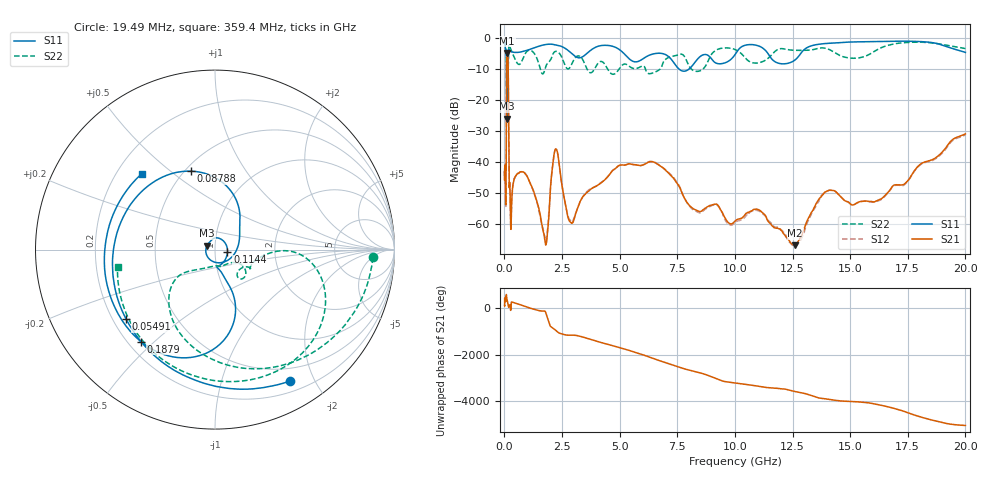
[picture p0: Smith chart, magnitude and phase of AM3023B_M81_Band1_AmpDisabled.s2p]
!Agilent Technologies,E8364B,MY43040894,A.07.50.67
!Agilent E8364B: A.07.50.67
!Date: Tuesday, October 27, 2020 10:39:40
!Correction: S11(Full 2 Port(1,2))
!S21(Full 2 Port(1,2))
!S12(Full 2 Port(1,2))
!S22(Full 2 Port(1,2))
!S2P File: Measurements: S11, S21, S12, S22:Log Frequency Sweep
# Hz S  dB  R 50
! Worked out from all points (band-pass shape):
!   3201 points, 10 MHz to 20 GHz, reference 50 ohm
!   highest |S21| = -4.93 dB at 122.5 MHz (marker M1); lowest = -66.9 dB at 12.62 GHz (marker M2)
!   |S21| within 3 dB of the highest: 96.52 MHz to 162.3 MHz (65.75 MHz wide, 50.8 % of centre)
!   lowest |S11| = -26.1 dB at 102.6 MHz (marker M3), VSWR 1.10, Z = 45.7 + j1.99 ohm
!   |S11| at or under -10 dB: 91.5 MHz to 160.5 MHz (68.95 MHz wide, 54.7 % of centre); 7.563 GHz to 8.025 GHz (461.9 MHz wide, 5.93 % of centre)
!   |S22| runs from -20.9 to -0.9 dB; largest |S21 - S12| = 0.012
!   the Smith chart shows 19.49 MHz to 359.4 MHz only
!   S11 on the Smith chart (normalised r, x): 19.49 MHz: 0.33, -1.67; 54.91 MHz: 0.25, -0.33; 87.88 MHz: 0.53, +0.59; 114.4 MHz: 1.15, -0.04; 187.9 MHz: 0.25, -0.45; 359.4 MHz: 0.30, +0.39
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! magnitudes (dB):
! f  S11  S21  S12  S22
! 10 MHz  -0.9  -44.5  -42.2  -1.0
! 19.49 MHz  -1.5  -42.8  -41.4  -1.1
! 35.55 MHz  -2.7  -41.9  -41.8  -1.5
! 54.91 MHz  -4.0  -53.5  -53.5  -2.4
! 78.78 MHz  -5.4  -41.7  -41.7  -4.9
! 87.88 MHz  -6.8  -21.0  -21.1  -9.2
! 102.6 MHz  -26.1  -6.0  -6.0  -20.0
! 114.4 MHz  -23.0  -5.0  -5.1  -15.3
! 122.5 MHz  -20.9  -4.9  -5.0  -13.0
! 126.1 MHz  -20.5  -4.9  -5.0  -13.4
! 161.4 MHz  -9.5  -7.6  -7.6  -12.3
! 187.9 MHz  -3.6  -30.0  -30.0  -2.7
! 278.8 MHz  -4.4  -61.5  -61.5  -3.7
! 359.4 MHz  -4.6  -47.9  -48.1  -5.2
! 447.2 MHz  -4.7  -45.2  -45.2  -6.7
! 1.59 GHz  -2.5  -58.7  -59.1  -10.8
! 1.829 GHz  -2.1  -65.9  -64.5  -8.7
! 2.222 GHz  -2.3  -35.9  -35.9  -4.4
! 2.893 GHz  -4.9  -59.6  -59.2  -8.9
! 5.639 GHz  -7.7  -40.9  -40.9  -9.9
! 12.62 GHz  -7.1  -66.9  -67.2  -4.0
! 20 GHz  -4.7  -31.0  -31.3  -3.5
